PROGRAM P_Prog5
VAR

	fbKL6401 					: FB_LON_KL6401;

	fbREAD_125		: FB_READ_125_SNVT_ph;
	fbSEND_125		: FB_SEND_125_SNVT_ph;

	fbREAD_126		: FB_READ_126_SNVT_ph_f;
	fbSEND_126		: FB_SEND_126_SNVT_ph_f;

	fbREAD_127		: FB_READ_127_SNVT_chlr_status;
	fbSEND_127		: FB_SEND_127_SNVT_chlr_status;

	fbREAD_128		: FB_READ_128_SNVT_tod_event;
	fbSEND_128		: FB_SEND_128_SNVT_tod_event;

	fbREAD_129		: FB_READ_129_SNVT_smo_obscur;
	fbSEND_129		: FB_SEND_129_SNVT_smo_obscur;

	fbREAD_130		: FB_READ_130_SNVT_fire_test;
	fbSEND_130		: FB_SEND_130_SNVT_fire_test;

	fbREAD_131		: FB_READ_131_SNVT_temp_ror;
	fbSEND_131		: FB_SEND_131_SNVT_temp_ror;

	fbREAD_132		: FB_READ_132_SNVT_fire_init;
	fbSEND_132		: FB_SEND_132_SNVT_fire_init;

	fbREAD_133		: FB_READ_133_SNVT_fire_indcte;
	fbSEND_133		: FB_SEND_133_SNVT_fire_indcte;

	fbREAD_134		: FB_READ_134_SNVT_time_zone;
	fbSEND_134		: FB_SEND_134_SNVT_time_zone;

	fbREAD_135		: FB_READ_135_SNVT_earth_pos;
	fbSEND_135		: FB_SEND_135_SNVT_earth_pos;

	fbREAD_136		: FB_READ_136_SNVT_reg_val;
	fbSEND_136		: FB_SEND_136_SNVT_reg_val;

	fbREAD_137		: FB_READ_137_SNVT_reg_val_ts;
	fbSEND_137		: FB_SEND_137_SNVT_reg_val_ts;

	fbREAD_138		: FB_READ_138_SNVT_volt_ac;
	fbSEND_138		: FB_SEND_138_SNVT_volt_ac;

	fbREAD_139		: FB_READ_139_SNVT_amp_ac;
	fbSEND_139		: FB_SEND_139_SNVT_amp_ac;

(*
	fbREAD_140		: FB_READ_109_SNVT_occupancy;
	fbSEND_140		: FB_SEND_109_SNVT_occupancy;

	fbREAD_141		: FB_READ_110_SNVT_area;
	fbSEND_141		: FB_SEND_110_SNVT_area;

	fbREAD_142		: FB_READ_111_SNVT_hvac_overid;
	fbSEND_142		: FB_SEND_111_SNVT_hvac_overid;
*)
	fbREAD_143		: FB_READ_143_SNVT_turbidity;
	fbSEND_143		: FB_SEND_143_SNVT_turbidity;

	fbREAD_144		: FB_READ_144_SNVT_turbidity_f;
	fbSEND_144		: FB_SEND_144_SNVT_turbidity_f;

	fbREAD_145		: FB_READ_145_SNVT_hvac_type;
	fbSEND_145		: FB_SEND_145_SNVT_hvac_type;

	fbREAD_146		: FB_READ_146_SNVT_elec_kwh_l;
	fbSEND_146		: FB_SEND_146_SNVT_elec_kwh_l;

	fbREAD_147		: FB_READ_147_SNVT_temp_diff_p;
	fbSEND_147		: FB_SEND_147_SNVT_temp_diff_p;

	fbREAD_148		: FB_READ_148_SNVT_ctrl_req;
	fbSEND_148		: FB_SEND_148_SNVT_ctrl_req;

	fbREAD_149		: FB_READ_149_SNVT_ctrl_resp;
	fbSEND_149		: FB_SEND_149_SNVT_ctrl_resp;

	fbREAD_150		: FB_READ_150_SNVT_ptz;
	fbSEND_150		: FB_SEND_150_SNVT_ptz;

	fbREAD_151		: FB_READ_151_SNVT_privacyzone;
	fbSEND_151		: FB_SEND_151_SNVT_privacyzone;

	fbREAD_152		: FB_READ_152_SNVT_pos_ctrl;
	fbSEND_152		: FB_SEND_152_SNVT_pos_ctrl;

	fbREAD_153		: FB_READ_153_SNVT_enthalpy;
	fbSEND_153		: FB_SEND_153_SNVT_enthalpy;

	fbREAD_154		: FB_READ_154_SNVT_gfci_status;
	fbSEND_154		: FB_SEND_154_SNVT_gfci_status;

	fbREAD_155		: FB_READ_155_SNVT_motor_state;
	fbSEND_155		: FB_SEND_155_SNVT_motor_state;

	fbREAD_156		: FB_READ_156_SNVT_pumpset_mn;
	fbSEND_156		: FB_SEND_156_SNVT_pumpset_mn;

	fbREAD_157		: FB_READ_157_SNVT_ex_control;
	fbSEND_157		: FB_SEND_157_SNVT_ex_control;

	fbREAD_158		: FB_READ_158_SNVT_pumpset_sn;
	fbSEND_158		: FB_SEND_158_SNVT_pumpset_sn;

END_VAR


fbKL6401(
	bDisabled:=FALSE ,
	stParameter_IN:=LON_IN_5 ,
	stParameter_OUT:=LON_OUT_5 ,
	stLON_Com:=stLON_Com_5,
	bReady=> ,
	eError=> ,
	stKL6401=> ,
	arrProgID=> ,
	arrNeuronID=> ,
	bBusy=> ,
	bError=> ,
	dwErrorKL=> ,
	bTimeOut=> ,
	byLONState=> );

(**)
fbREAD_125(
	wNVIndex:=0 ,

	bDisabled:= ,
	stLON_Com:=stLON_Com_5,
	rValue=> ,
	bNewData=> ,
	bError=> ,
	eError=> );
fbREAD_125.rValue;
fbREAD_125.bError;
fbREAD_125.eError;

fbSEND_125.rValue;
fbSEND_125.bStart;
fbSEND_125.bError;
fbSEND_125.eError;
fbSEND_125.bBusy;
fbSEND_125.dwErrorKL;

fbSEND_125.bAuto;
fbSEND_125.bSendInit;
fbSEND_125.tMinSendTime;
fbSEND_125.tMaxSendTime;
fbSEND_125.rValueLimit;

fbSEND_125(
	wNVIndex:=1 ,
	bStart:= ,
	rValue:= ,
	bDisabled:= ,
	stLON_Com:=stLON_Com_5,
	bError=> ,
	eError=> );
fbSEND_125.bStart:=FALSE;

(**)
fbREAD_126(
	wNVIndex:=2 ,
	bDisabled:= ,
	stLON_Com:=stLON_Com_5,
	rValue=> ,
	bNewData=> ,
	bError=> ,
	eError=> );
fbREAD_126.rValue;
fbREAD_126.bError;
fbREAD_126.eError;

fbSEND_126.rValue;
fbSEND_126.bStart;
fbSEND_126.bError;
fbSEND_126.eError;
fbSEND_126.bBusy;
fbSEND_126.dwErrorKL;

fbSEND_126.bAuto;
fbSEND_126.bSendInit;
fbSEND_126.tMinSendTime;
fbSEND_126.tMaxSendTime;
fbSEND_126.rValueLimit;

fbSEND_126(
	wNVIndex:=3 ,
	bStart:= ,
	rValue:= ,
	bDisabled:= ,
	stLON_Com:=stLON_Com_5,
	bError=> ,
	eError=> );
fbSEND_126.bStart:=FALSE;

(**)
fbREAD_127(
	wNVIndex:=4 ,
	bDisabled:= ,
	stLON_Com:=stLON_Com_5,
	stValue=> ,
	bNewData=> ,
	bError=> ,
	eError=> );
fbREAD_127.stValue;
fbREAD_127.bError;
fbREAD_127.eError;

fbSEND_127.stValue;
fbSEND_127.bStart;
fbSEND_127.bError;
fbSEND_127.eError;
fbSEND_127.bBusy;
fbSEND_127.dwErrorKL;

fbSEND_127.bAuto;
fbSEND_127.bSendInit;
fbSEND_127.tMinSendTime;
fbSEND_127.tMaxSendTime;

fbSEND_127(
	wNVIndex:=5 ,
	bStart:= ,
	stValue:= ,
	bDisabled:= ,
	stLON_Com:=stLON_Com_5,
	bError=> ,
	eError=> );
fbSEND_127.bStart:=FALSE;

(**)
fbREAD_128(
	wNVIndex:=6 ,
	bDisabled:= ,
	stLON_Com:=stLON_Com_5,
	stValue=> ,
	bNewData=> ,
	bError=> ,
	eError=> );
fbREAD_128.stValue;
fbREAD_128.bError;
fbREAD_128.eError;

fbSEND_128.stValue;
fbSEND_128.bStart;
fbSEND_128.bError;
fbSEND_128.eError;
fbSEND_128.bBusy;
fbSEND_128.dwErrorKL;

fbSEND_128.bAuto;
fbSEND_128.bSendInit;
fbSEND_128.tMinSendTime;
fbSEND_128.tMaxSendTime;

fbSEND_128(
	wNVIndex:=7 ,
	bStart:= ,
	stValue:= ,
	bDisabled:= ,
	stLON_Com:=stLON_Com_5,
	bError=> ,
	eError=> );
fbSEND_128.bStart:=FALSE;

(**)
fbREAD_129(
	wNVIndex:=8 ,
	bDisabled:= ,
	stLON_Com:=stLON_Com_5,
	rValue=> ,
	bNewData=> ,
	bError=> ,
	eError=> );
fbREAD_129.rValue;
fbREAD_129.bError;
fbREAD_129.eError;

fbSEND_129.rValue;
fbSEND_129.bStart;
fbSEND_129.bError;
fbSEND_129.eError;
fbSEND_129.bBusy;
fbSEND_129.dwErrorKL;

fbSEND_129.bAuto;
fbSEND_129.bSendInit;
fbSEND_129.tMinSendTime;
fbSEND_129.tMaxSendTime;
fbSEND_129.rValueLimit;

fbSEND_129(
	wNVIndex:=9 ,
	bStart:= ,
	rValue:= ,
	bDisabled:= ,
	stLON_Com:=stLON_Com_5,
	bError=> ,
	eError=> );
fbSEND_129.bStart:=FALSE;

(**)
fbREAD_130(
	wNVIndex:=10 ,
	bDisabled:= ,
	stLON_Com:=stLON_Com_5,
	eValue=> ,
	bNewData=> ,
	bError=> ,
	eError=> );
fbREAD_130.eValue;
fbREAD_130.bError;
fbREAD_130.eError;

fbSEND_130.eValue;
fbSEND_130.bStart;
fbSEND_130.bError;
fbSEND_130.eError;
fbSEND_130.bBusy;
fbSEND_130.dwErrorKL;

fbSEND_130.bAuto;
fbSEND_130.bSendInit;
fbSEND_130.tMinSendTime;
fbSEND_130.tMaxSendTime;

fbSEND_130(
	wNVIndex:=11 ,
	bStart:= ,
	eValue:= ,
	bDisabled:= ,
	stLON_Com:=stLON_Com_5,
	bError=> ,
	eError=> );
fbSEND_130.bStart:=FALSE;

(**)
fbREAD_131(
	wNVIndex:=12 ,
	bDisabled:= ,
	stLON_Com:=stLON_Com_5,
	rValue=> ,
	bNewData=> ,
	bError=> ,
	eError=> );
fbREAD_131.rValue;
fbREAD_131.bError;
fbREAD_131.eError;

fbSEND_131.rValue;
fbSEND_131.bStart;
fbSEND_131.bError;
fbSEND_131.eError;
fbSEND_131.bBusy;
fbSEND_131.dwErrorKL;

fbSEND_131.bAuto;
fbSEND_131.bSendInit;
fbSEND_131.tMinSendTime;
fbSEND_131.tMaxSendTime;
fbSEND_131.rValueLimit;

fbSEND_131(
	wNVIndex:=13 ,
	bStart:= ,
	rValue:= ,
	bDisabled:= ,
	stLON_Com:=stLON_Com_5,
	bError=> ,
	eError=> );
fbSEND_131.bStart:=FALSE;

(**)
fbREAD_132(
	wNVIndex:=14 ,
	bDisabled:= ,
	stLON_Com:=stLON_Com_5,
	eValue=> ,
	bNewData=> ,
	bError=> ,
	eError=> );
fbREAD_132.eValue;
fbREAD_132.bError;
fbREAD_132.eError;

fbSEND_132.eValue;
fbSEND_132.bStart;
fbSEND_132.bError;
fbSEND_132.eError;
fbSEND_132.bBusy;
fbSEND_132.dwErrorKL;


fbSEND_132.bAuto;
fbSEND_132.bSendInit;
fbSEND_132.tMinSendTime;
fbSEND_132.tMaxSendTime;

fbSEND_132(
	wNVIndex:=15 ,
	bStart:= ,
	eValue:= ,
	bDisabled:= ,
	stLON_Com:=stLON_Com_5,
	bError=> ,
	eError=> );
fbSEND_132.bStart:=FALSE;

(**)
fbREAD_133(
	wNVIndex:=16 ,
	bDisabled:= ,
	stLON_Com:=stLON_Com_5,
	eValue=> ,
	bNewData=> ,
	bError=> ,
	eError=> );
fbREAD_133.eValue;
fbREAD_133.bError;
fbREAD_133.eError;

fbSEND_133.eValue;
fbSEND_133.bStart;
fbSEND_133.bError;
fbSEND_133.eError;
fbSEND_133.bBusy;
fbSEND_133.dwErrorKL;

fbSEND_133.bAuto;
fbSEND_133.bSendInit;
fbSEND_133.tMinSendTime;
fbSEND_133.tMaxSendTime;

fbSEND_133(
	wNVIndex:=17 ,
	bStart:= ,
	eValue:= ,
	bDisabled:= ,
	stLON_Com:=stLON_Com_5,
	bError=> ,
	eError=> );
fbSEND_133.bStart:=FALSE;

(**)
fbREAD_134(
	wNVIndex:=18 ,
	bDisabled:= ,
	stLON_Com:=stLON_Com_5,
	stValue=> ,
	bNewData=> ,
	bError=> ,
	eError=> );
fbREAD_134.stValue;
fbREAD_134.bError;
fbREAD_134.eError;

fbSEND_134.stValue;
fbSEND_134.bStart;
fbSEND_134.bError;
fbSEND_134.eError;
fbSEND_134.bBusy;
fbSEND_134.dwErrorKL;

fbSEND_134.bAuto;
fbSEND_134.bSendInit;
fbSEND_134.tMinSendTime;
fbSEND_134.tMaxSendTime;

fbSEND_134(
	wNVIndex:=19 ,
	bStart:= ,
	stValue:= ,
	bDisabled:= ,
	stLON_Com:=stLON_Com_5,
	bError=> ,
	eError=> );
fbSEND_134.bStart:=FALSE;

(**)
fbREAD_135(
	wNVIndex:=20 ,
	bDisabled:= ,
	stLON_Com:=stLON_Com_5,
	stValue=> ,
	bNewData=> ,
	bError=> ,
	eError=> );
fbREAD_135.stValue;
fbREAD_135.bError;
fbREAD_135.eError;

fbSEND_135.stValue;
fbSEND_135.bStart;
fbSEND_135.bError;
fbSEND_135.eError;
fbSEND_135.bBusy;
fbSEND_135.dwErrorKL;

fbSEND_135.bAuto;
fbSEND_135.bSendInit;
fbSEND_135.tMinSendTime;
fbSEND_135.tMaxSendTime;

fbSEND_135(
	wNVIndex:=21 ,
	bStart:= ,
	stValue:= ,
	bDisabled:= ,
	stLON_Com:=stLON_Com_5,
	bError=> ,
	eError=> );
fbSEND_135.bStart:=FALSE;

(**)
fbREAD_136(
	wNVIndex:=22 ,
	bDisabled:= ,
	stLON_Com:=stLON_Com_5,
	stValue=> ,
	bNewData=> ,
	bError=> ,
	eError=> );
fbREAD_136.stValue;
fbREAD_136.bError;
fbREAD_136.eError;

fbSEND_136.stValue;
fbSEND_136.bStart;
fbSEND_136.bError;
fbSEND_136.eError;
fbSEND_136.bBusy;
fbSEND_136.dwErrorKL;

fbSEND_136.bAuto;
fbSEND_136.bSendInit;
fbSEND_136.tMinSendTime;
fbSEND_136.tMaxSendTime;

fbSEND_136(
	wNVIndex:=23 ,
	bStart:= ,
	stValue:= ,
	bDisabled:= ,
	stLON_Com:=stLON_Com_5,
	bError=> ,
	eError=> );
fbSEND_136.bStart:=FALSE;

(**)
fbREAD_137(
	wNVIndex:=24 ,
	bDisabled:= ,
	stLON_Com:=stLON_Com_5,
	stValue=> ,
	bNewData=> ,
	bError=> ,
	eError=> );
fbREAD_137.stValue;
fbREAD_137.bError;
fbREAD_137.eError;

fbSEND_137.stValue;
fbSEND_137.bStart;
fbSEND_137.bError;
fbSEND_137.eError;
fbSEND_137.bBusy;
fbSEND_137.dwErrorKL;

fbSEND_137.bAuto;
fbSEND_137.bSendInit;
fbSEND_137.tMinSendTime;
fbSEND_137.tMaxSendTime;

fbSEND_137(
	wNVIndex:=25 ,
	bStart:= ,
	stValue:= ,
	bDisabled:= ,
	stLON_Com:=stLON_Com_5,
	bError=> ,
	eError=> );
fbSEND_137.bStart:=FALSE;

(**)
fbREAD_138(
	wNVIndex:=26 ,
	bDisabled:= ,
	stLON_Com:=stLON_Com_5,
	uiValue=> ,
	bNewData=> ,
	bError=> ,
	eError=> );
fbREAD_138.uiValue;
fbREAD_138.bError;
fbREAD_138.eError;

fbSEND_138.uiValue;
fbSEND_138.bStart;
fbSEND_138.bError;
fbSEND_138.eError;
fbSEND_138.bBusy;
fbSEND_138.dwErrorKL;

fbSEND_138.bAuto;
fbSEND_138.bSendInit;
fbSEND_138.tMinSendTime;
fbSEND_138.tMaxSendTime;
fbSEND_138.uiValueLimit;

fbSEND_138(
	wNVIndex:=27 ,
	bStart:= ,
	uiValue:= ,
	bDisabled:= ,
	stLON_Com:=stLON_Com_5,
	bError=> ,
	eError=> );
fbSEND_138.bStart:=FALSE;

(**)
fbREAD_139(
	wNVIndex:=28 ,
	bDisabled:= ,
	stLON_Com:=stLON_Com_5,
	uiValue=> ,
	bNewData=> ,
	bError=> ,
	eError=> );
fbREAD_139.uiValue;
fbREAD_139.bError;
fbREAD_139.eError;

fbSEND_139.uiValue;
fbSEND_139.bStart;
fbSEND_139.bError;
fbSEND_139.eError;
fbSEND_139.bBusy;
fbSEND_139.dwErrorKL;

fbSEND_139.bAuto;
fbSEND_139.bSendInit;
fbSEND_139.tMinSendTime;
fbSEND_139.tMaxSendTime;
fbSEND_139.uiValueLimit;

fbSEND_139(
	wNVIndex:=29 ,
	bStart:= ,
	uiValue:= ,
	bDisabled:= ,
	stLON_Com:=stLON_Com_5,
	bError=> ,
	eError=> );
fbSEND_139.bStart:=FALSE;

(**)
fbREAD_143(
	wNVIndex:=30 ,
	bDisabled:= ,
	stLON_Com:=stLON_Com_5,
	rValue=> ,
	bNewData=> ,
	bError=> ,
	eError=> );
fbREAD_143.rValue;
fbREAD_143.bError;
fbREAD_143.eError;

fbSEND_143.rValue;
fbSEND_143.bStart;
fbSEND_143.bError;
fbSEND_143.eError;
fbSEND_143.bBusy;
fbSEND_143.dwErrorKL;

fbSEND_143.bAuto;
fbSEND_143.bSendInit;
fbSEND_143.tMinSendTime;
fbSEND_143.tMaxSendTime;
fbSEND_143.rValueLimit;

fbSEND_143(
	wNVIndex:=31 ,
	bStart:= ,
	rValue:= ,
	bDisabled:= ,
	stLON_Com:=stLON_Com_5,
	bError=> ,
	eError=> );
fbSEND_143.bStart:=FALSE;

(**)
fbREAD_144(
	wNVIndex:=32 ,
	bDisabled:= ,
	stLON_Com:=stLON_Com_5,
	rValue=> ,
	bNewData=> ,
	bError=> ,
	eError=> );
fbREAD_144.rValue;
fbREAD_144.bError;
fbREAD_144.eError;

fbSEND_144.rValue;
fbSEND_144.bStart;
fbSEND_144.bError;
fbSEND_144.eError;
fbSEND_144.bBusy;
fbSEND_144.dwErrorKL;

fbSEND_144.bAuto;
fbSEND_144.bSendInit;
fbSEND_144.tMinSendTime;
fbSEND_144.tMaxSendTime;
fbSEND_144.rValueLimit;

fbSEND_144(
	wNVIndex:=33 ,
	bStart:= ,
	rValue:= ,
	bDisabled:= ,
	stLON_Com:=stLON_Com_5,
	bError=> ,
	eError=> );
fbSEND_144.bStart:=FALSE;

(**)
fbREAD_145(
	wNVIndex:=34 ,
	bDisabled:= ,
	stLON_Com:=stLON_Com_5,
	eValue=> ,
	bNewData=> ,
	bError=> ,
	eError=> );
fbREAD_145.eValue;
fbREAD_145.bError;
fbREAD_145.eError;

fbSEND_145.eValue;
fbSEND_145.bStart;
fbSEND_145.bError;
fbSEND_145.eError;
fbSEND_145.bBusy;
fbSEND_145.dwErrorKL;

fbSEND_145.bAuto;
fbSEND_145.bSendInit;
fbSEND_145.tMinSendTime;
fbSEND_145.tMaxSendTime;

fbSEND_145(
	wNVIndex:=35 ,
	bStart:= ,
	eValue:= ,
	bDisabled:= ,
	stLON_Com:=stLON_Com_5,
	bError=> ,
	eError=> );
fbSEND_145.bStart:=FALSE;

(**)
fbREAD_146(
	wNVIndex:=36 ,
	bDisabled:= ,
	stLON_Com:=stLON_Com_5,
	lrValue=> ,
	bNewData=> ,
	bError=> ,
	eError=> );
fbREAD_146.lrValue;
fbREAD_146.bError;
fbREAD_146.eError;

fbSEND_146.lrValue;
fbSEND_146.bStart;
fbSEND_146.bError;
fbSEND_146.eError;
fbSEND_146.bBusy;
fbSEND_146.dwErrorKL;

fbSEND_146.bAuto;
fbSEND_146.bSendInit;
fbSEND_146.tMinSendTime;
fbSEND_146.tMaxSendTime;
fbSEND_146.lrValueLimit;

fbSEND_146(
	wNVIndex:=37 ,
	bStart:= ,
	lrValue:= ,
	bDisabled:= ,
	stLON_Com:=stLON_Com_5,
	bError=> ,
	eError=> );
fbSEND_146.bStart:=FALSE;

(**)
fbREAD_147(
	wNVIndex:=38 ,
	bDisabled:= ,
	stLON_Com:=stLON_Com_5,
	rValue=> ,
	bNewData=> ,
	bError=> ,
	eError=> );
fbREAD_147.rValue;
fbREAD_147.bError;
fbREAD_147.eError;

fbSEND_147.rValue;
fbSEND_147.bStart;
fbSEND_147.bError;
fbSEND_147.eError;
fbSEND_147.bBusy;
fbSEND_147.dwErrorKL;

fbSEND_147.bAuto;
fbSEND_147.bSendInit;
fbSEND_147.tMinSendTime;
fbSEND_147.tMaxSendTime;
fbSEND_147.rValueLimit;

fbSEND_147(
	wNVIndex:=39 ,
	bStart:= ,
	rValue:= ,
	bDisabled:= ,
	stLON_Com:=stLON_Com_5,
	bError=> ,
	eError=> );
fbSEND_147.bStart:=FALSE;

(**)
fbREAD_148(
	wNVIndex:=40 ,
	bDisabled:= ,
	stLON_Com:=stLON_Com_5,
	stValue=> ,
	bNewData=> ,
	bError=> ,
	eError=> );
fbREAD_148.stValue;
fbREAD_148.bError;
fbREAD_148.eError;

fbSEND_148.stValue;
fbSEND_148.bStart;
fbSEND_148.bError;
fbSEND_148.eError;
fbSEND_148.bBusy;
fbSEND_148.dwErrorKL;

fbSEND_148.bAuto;
fbSEND_148.bSendInit;
fbSEND_148.tMinSendTime;
fbSEND_148.tMaxSendTime;

fbSEND_148(
	wNVIndex:=41 ,
	bStart:= ,
	stValue:= ,
	bDisabled:= ,
	stLON_Com:=stLON_Com_5,
	bError=> ,
	eError=> );
fbSEND_148.bStart:=FALSE;

(**)
fbREAD_149(
	wNVIndex:=42 ,
	bDisabled:= ,
	stLON_Com:=stLON_Com_5,
	stValue=> ,
	bNewData=> ,
	bError=> ,
	eError=> );
fbREAD_149.stValue;
fbREAD_149.bError;
fbREAD_149.eError;

fbSEND_149.stValue;
fbSEND_149.bStart;
fbSEND_149.bError;
fbSEND_149.eError;
fbSEND_149.bBusy;
fbSEND_149.dwErrorKL;

fbSEND_149.bAuto;
fbSEND_149.bSendInit;
fbSEND_149.tMinSendTime;
fbSEND_149.tMaxSendTime;

fbSEND_149(
	wNVIndex:=43 ,
	bStart:= ,
	stValue:= ,
	bDisabled:= ,
	stLON_Com:=stLON_Com_5,
	bError=> ,
	eError=> );
fbSEND_149.bStart:=FALSE;

(**)
fbREAD_150(
	wNVIndex:=44 ,
	bDisabled:= ,
	stLON_Com:=stLON_Com_5,
	stValue=> ,
	bNewData=> ,
	bError=> ,
	eError=> );
fbREAD_150.stValue;
fbREAD_150.bError;
fbREAD_150.eError;

fbSEND_150.stValue;
fbSEND_150.bStart;
fbSEND_150.bError;
fbSEND_150.eError;
fbSEND_150.bBusy;
fbSEND_150.dwErrorKL;

fbSEND_150.bAuto;
fbSEND_150.bSendInit;
fbSEND_150.tMinSendTime;
fbSEND_150.tMaxSendTime;

fbSEND_150(
	wNVIndex:=45 ,
	bStart:= ,
	stValue:= ,
	bDisabled:= ,
	stLON_Com:=stLON_Com_5,
	bError=> ,
	eError=> );
fbSEND_150.bStart:=FALSE;

(**)
fbREAD_151(
	wNVIndex:=46 ,
	bDisabled:= ,
	stLON_Com:=stLON_Com_5,
	stValue=> ,
	bNewData=> ,
	bError=> ,
	eError=> );
fbREAD_151.stValue;
fbREAD_151.bError;
fbREAD_151.eError;

fbSEND_151.stValue;
fbSEND_151.bStart;
fbSEND_151.bError;
fbSEND_151.eError;
fbSEND_151.bBusy;
fbSEND_151.dwErrorKL;

fbSEND_151.bAuto;
fbSEND_151.bSendInit;
fbSEND_151.tMinSendTime;
fbSEND_151.tMaxSendTime;

fbSEND_151(
	wNVIndex:=47 ,
	bStart:= ,
	stValue:= ,
	bDisabled:= ,
	stLON_Com:=stLON_Com_5,
	bError=> ,
	eError=> );
fbSEND_151.bStart:=FALSE;

(**)
fbREAD_152(
	wNVIndex:=48 ,
	bDisabled:= ,
	stLON_Com:=stLON_Com_5,
	stValue=> ,
	bNewData=> ,
	bError=> ,
	eError=> );
fbREAD_152.stValue;
fbREAD_152.bError;
fbREAD_152.eError;

fbSEND_152.stValue;
fbSEND_152.bStart;
fbSEND_152.bError;
fbSEND_152.eError;
fbSEND_152.bBusy;
fbSEND_152.dwErrorKL;

fbSEND_152.bAuto;
fbSEND_152.bSendInit;
fbSEND_152.tMinSendTime;
fbSEND_152.tMaxSendTime;

fbSEND_152(
	wNVIndex:=49 ,
	bStart:= ,
	stValue:= ,
	bDisabled:= ,
	stLON_Com:=stLON_Com_5,
	bError=> ,
	eError=> );
fbSEND_152.bStart:=FALSE;

(**)
fbREAD_153(
	wNVIndex:=50 ,
	bDisabled:= ,
	stLON_Com:=stLON_Com_5,
	rValue=> ,
	bNewData=> ,
	bError=> ,
	eError=> );
fbREAD_153.rValue;
fbREAD_153.bError;
fbREAD_153.eError;

fbSEND_153.rValue;
fbSEND_153.bStart;
fbSEND_153.bError;
fbSEND_153.eError;
fbSEND_153.bBusy;
fbSEND_153.dwErrorKL;

fbSEND_153.bAuto;
fbSEND_153.bSendInit;
fbSEND_153.tMinSendTime;
fbSEND_153.tMaxSendTime;
fbSEND_153.rValueLimit;

fbSEND_153(
	wNVIndex:=51 ,
	bStart:= ,
	rValue:= ,
	bDisabled:= ,
	stLON_Com:=stLON_Com_5,
	bError=> ,
	eError=> );
fbSEND_153.bStart:=FALSE;

(**)
fbREAD_154(
	wNVIndex:=52 ,
	bDisabled:= ,
	stLON_Com:=stLON_Com_5,
	eValue=> ,
	bNewData=> ,
	bError=> ,
	eError=> );
fbREAD_154.eValue;
fbREAD_154.bError;
fbREAD_154.eError;

fbSEND_154.eValue;
fbSEND_154.bStart;
fbSEND_154.bError;
fbSEND_154.eError;
fbSEND_154.bBusy;
fbSEND_154.dwErrorKL;

fbSEND_154.bAuto;
fbSEND_154.bSendInit;
fbSEND_154.tMinSendTime;
fbSEND_154.tMaxSendTime;

fbSEND_154(
	wNVIndex:=53 ,
	bStart:= ,
	eValue:= ,
	bDisabled:= ,
	stLON_Com:=stLON_Com_5,
	bError=> ,
	eError=> );
fbSEND_154.bStart:=FALSE;

(**)
fbREAD_155(
	wNVIndex:=54 ,
	bDisabled:= ,
	stLON_Com:=stLON_Com_5,
	eValue=> ,
	bNewData=> ,
	bError=> ,
	eError=> );
fbREAD_155.eValue;
fbREAD_155.bError;
fbREAD_155.eError;

fbSEND_155.eValue;
fbSEND_155.bStart;
fbSEND_155.bError;
fbSEND_155.eError;
fbSEND_155.bBusy;
fbSEND_155.dwErrorKL;

fbSEND_155.bAuto;
fbSEND_155.bSendInit;
fbSEND_155.tMinSendTime;
fbSEND_155.tMaxSendTime;

fbSEND_155(
	wNVIndex:=55 ,
	bStart:= ,
	eValue:= ,
	bDisabled:= ,
	stLON_Com:=stLON_Com_5,
	bError=> ,
	eError=> );
fbSEND_155.bStart:=FALSE;

(**)
fbREAD_156(
	wNVIndex:=56 ,
	bDisabled:= ,
	stLON_Com:=stLON_Com_5,
	stValue=> ,
	bNewData=> ,
	bError=> ,
	eError=> );
fbREAD_156.stValue;
fbREAD_156.bError;
fbREAD_156.eError;

fbSEND_156.stValue;
fbSEND_156.bStart;
fbSEND_156.bError;
fbSEND_156.eError;
fbSEND_156.bBusy;
fbSEND_156.dwErrorKL;

fbSEND_156.bAuto;
fbSEND_156.bSendInit;
fbSEND_156.tMinSendTime;
fbSEND_156.tMaxSendTime;

fbSEND_156(
	wNVIndex:=57 ,
	bStart:= ,
	stValue:= ,
	bDisabled:= ,
	stLON_Com:=stLON_Com_5,
	bError=> ,
	eError=> );
fbSEND_156.bStart:=FALSE;

(**)
fbREAD_157(
	wNVIndex:=58 ,
	bDisabled:= ,
	stLON_Com:=stLON_Com_5,
	stValue=> ,
	bNewData=> ,
	bError=> ,
	eError=> );
fbREAD_157.stValue;
fbREAD_157.bError;
fbREAD_157.eError;

fbSEND_157.stValue;
fbSEND_157.bStart;
fbSEND_157.bError;
fbSEND_157.eError;
fbSEND_157.bBusy;
fbSEND_157.dwErrorKL;

fbSEND_157.bAuto;
fbSEND_157.bSendInit;
fbSEND_157.tMinSendTime;
fbSEND_157.tMaxSendTime;

fbSEND_157(
	wNVIndex:=59 ,
	bStart:= ,
	stValue:= ,
	bDisabled:= ,
	stLON_Com:=stLON_Com_5,
	bError=> ,
	eError=> );
fbSEND_157.bStart:=FALSE;

(**)
fbREAD_158(
	wNVIndex:=60 ,
	bDisabled:= ,
	stLON_Com:=stLON_Com_5,
	stValue=> ,
	bNewData=> ,
	bError=> ,
	eError=> );
fbREAD_158.stValue;
fbREAD_158.bError;
fbREAD_158.eError;

fbSEND_158.stValue;
fbSEND_158.bStart;
fbSEND_158.bError;
fbSEND_158.eError;
fbSEND_158.bBusy;
fbSEND_158.dwErrorKL;

fbSEND_158.bAuto;
fbSEND_158.bSendInit;
fbSEND_158.tMinSendTime;
fbSEND_158.tMaxSendTime;

fbSEND_158(
	wNVIndex:=61 ,
	bStart:= ,
	stValue:= ,
	bDisabled:= ,
	stLON_Com:=stLON_Com_5,
	bError=> ,
	eError=> );
fbSEND_158.bStart:=FALSE;

END_PROGRAM
